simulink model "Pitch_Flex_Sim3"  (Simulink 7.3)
settings: Solver=ode3  StartTime=0.0  StopTime=120  FixedStep=0.04  RelTol=1e-3
InitFcn:
  | r2d= 180/pi; d2r=1/r2d; Ts=0.04;
  | [Apf,Bpf,Cpf,Dpf]= pitch_vehi_flex;              % Shuttle Ascent, Max_Q, T=55 sec, Flex Pitch Vehicle with Slosh and TWD
  | [Aac,Bac,Cac,Dac]= ssme_actuator;                % Shuttle Main Engine Actuator
  | [Asb,Bsb,Csb,Dsb]= srb_actuator;                 % Solid Rocket Booster Actuator
  | [Afc,Bfc,Cfc,Dfc]= pitch_fcs;                    % Pitch Axis Discrete FCS
  | [Apl,Bpl,Cpl,Dpl]= pitch_plant_s;                % Pitch Plant (Flex Vehicle, Actuators, TVC, TWD)
  | [Apz,Bpz,Cpz,Dpz]= pitch_plant_z;                % Pitch Plant Discrete
  | [Aol,Bol,Col,Dol]= open_loop;                    % Open-Loop Pitch (Plant Model + Controller)
  | [Acl,Bcl,Ccl,Dcl]= closed_loop;                  % Closed Loop (Plant Model + Controller)
StopFcn:
  | pl2
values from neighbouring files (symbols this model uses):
  Acl = [    [closed_loop.m]
  Bcl = [    [closed_loop.m]
  Ccl = [    [closed_loop.m]
  Dcl = [    [closed_loop.m]

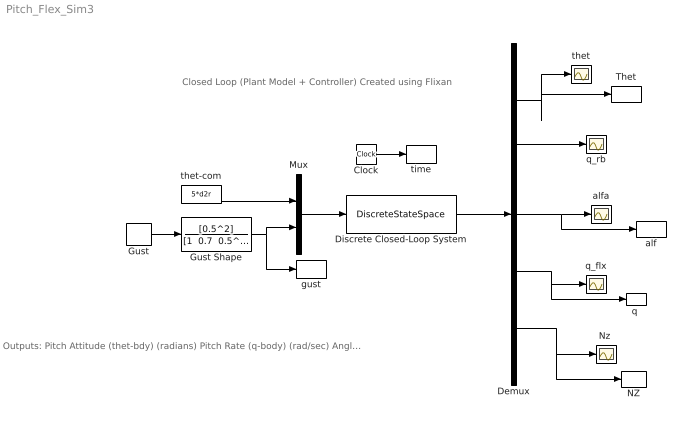
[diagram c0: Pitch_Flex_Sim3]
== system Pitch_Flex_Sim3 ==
  note: Outputs: Pitch Attitude (thet-bdy) (radians) Pitch Rate (q-body) (rad/sec) Angle of attack, alfa, (radians) Rate-Gyro # 2, Pitch Rate (Body) (rad/sec) Accelerom # 2, (along Z), (ft/sec^2) Translat. Acceleration
  note: Closed Loop (Plant Model + Controller) Created using Flixan
  Clock : Clock
  Demux : Demux  Outputs=5
  Discrete Closed-Loop System : DiscreteStateSpace  A=Acl  B=Bcl  C=Ccl  D=Dcl  SampleTime=0.04
  Gust : DiscretePulseGenerator  PulseType=Time based  Amplitude=30  Period=200  PulseWidth=5  PhaseDelay=0.2  SampleTime=1
  Gust Shape : TransferFcn  Numerator=[0.5^2]  Denominator="[1  0.7  0.5^2]"
  Mux : Mux  Inputs=2
  NZ : ToWorkspace  VariableName=Nz  SampleTime=-1  SaveFormat=Array
  "Nz " : Scope
  Thet : ToWorkspace  VariableName=theta  SampleTime=-1  SaveFormat=Array
  alf : ToWorkspace  VariableName=alpha  SampleTime=-1  SaveFormat=Array
  alfa : Scope
  gust : ToWorkspace  VariableName=Gust  SampleTime=-1  SaveFormat=Array
  "q " : ToWorkspace  VariableName=q  SampleTime=-1  SaveFormat=Array
  q_flx : Scope
  q_rb : Scope
  thet : Scope
  thet-com : Constant  Value=5*d2r  OutDataType=sfix(16)  OutScaling=2^0
  time : ToWorkspace  VariableName=time  SampleTime=-1  SaveFormat=Array
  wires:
  Mux/1 -> Discrete Closed-Loop System/1
  Demux/2 -> q_rb/1
  Demux/4 -> q_flx/1, "q "/1
  Discrete Closed-Loop System/1 -> Demux/1
  Demux/1 -> thet/1, Thet/1
  Demux/3 -> alfa/1, alf/1
  Demux/5 -> "Nz "/1, NZ/1
  thet-com/1 -> Mux/1
  Gust/1 -> Gust Shape/1
  Clock/1 -> time/1
  Gust Shape/1 -> Mux/2, gust/1
